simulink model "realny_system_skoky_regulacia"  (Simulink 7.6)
settings: Solver=ode4  StartTime=0.0  StopTime=150  FixedStep=0.2  RelTol=1e-3
undefined symbols (not defined in the file or in its folder): ABOVE_NORMAL_PRIORITY, COM3, D, I, lightbulb

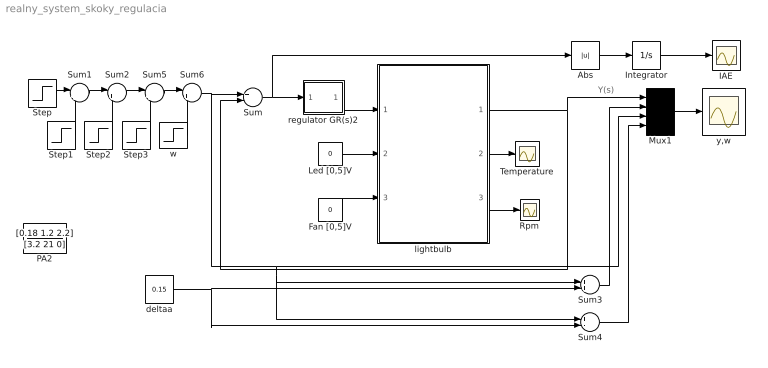
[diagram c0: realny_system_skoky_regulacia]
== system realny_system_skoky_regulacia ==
  note: Y(s)
  Abs : Abs
  Fan [0,5]V : Constant  Value=0
  IAE : Scope
  Integrator : Integrator
  Led [0,5]V : Constant  Value=0
  Mux1 : Mux
  PA2 : TransferFcn  Numerator=[0.18 1.2 2.2]  Denominator=[3.2 21 0]
  Rpm : Scope
  Step : Step  Time=0  After=11  SampleTime=0
  Step1 : Step  Time=30  After=30  SampleTime=0
  Step2 : Step  Time=60  After=-11  SampleTime=0
  Step3 : Step  Time=90  After=-25  SampleTime=0
  Sum : Sum  Inputs=+-
  Sum{1..2,5..6} (4 alike) : Sum  Inputs=|++
  Sum3 : Sum
  Sum4 : Sum  Inputs=+-
  Temperature : Scope
  deltaa : Constant  Value=0.15
  lightbulb : Subsystem  AncestorBlock=lightbulb/lightbulb
  regulator GR(s)2 : Subsystem  mask(PID Controller){P=0.059142,  I=0.059142/0.5163,  D=0}
      mask prompts: P "Proportional";  I "Integral";  D "Derivative"
      mask help: Enter expressions for proportional, integral, and derivative terms. P+I/s+Ds
  w : Step  Time=120  After=17  SampleTime=0
  y,w : Scope
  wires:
  Sum6/1 -> Sum3/1, Sum4/1, Mux1/3, Sum/1
  regulator GR(s)2/1(Out_1) -> lightbulb/1(bulb)
  Mux1/1 -> y,w/1
  deltaa/1 -> Sum3/2, Sum4/2
  Sum3/1 -> Mux1/2
  Sum4/1 -> Mux1/4
  lightbulb/1(light) -> Sum/2, Mux1/1
  Step1/1 -> Sum1/2
  Step/1 -> Sum1/1
  Step2/1 -> Sum2/2
  Step3/1 -> Sum5/2
  Sum2/1 -> Sum5/1
  Sum1/1 -> Sum2/1
  Sum5/1 -> Sum6/1
  w/1 -> Sum6/2
  Fan [0,5]V/1 -> lightbulb/3(fan)
  lightbulb/2(temperature) -> Temperature/1
  lightbulb/3(rpm) -> Rpm/1
  Led [0,5]V/1 -> lightbulb/2(led)
  Integrator/1 -> IAE/1
  Abs/1 -> Integrator/1
  Sum/1 -> regulator GR(s)2/1(In_1), Abs/1

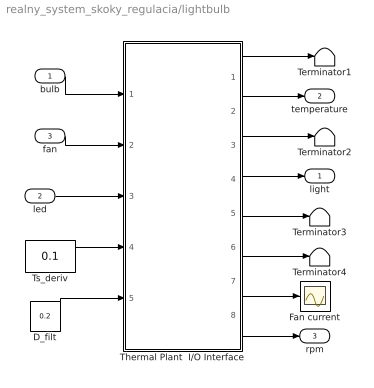
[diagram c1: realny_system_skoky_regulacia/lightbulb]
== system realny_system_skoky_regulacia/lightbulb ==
  bulb : Inport
  led : Inport  Port=2
  fan : Inport  Port=3
  D_filt : Constant  Value=0.2
  Fan current : Scope
  Terminator{1..4} (4 alike) : Terminator
  Thermal Plant  I/O Interface : Subsystem  mask{Ts=0.2}
      mask prompts: Ts "Sample time (s)"
      mask init:
      | set_param(bdroot,'FixedStep',num2str(Ts));
  Ts_deriv : Constant  Value=0.1
  light : Outport
  temperature : Outport  Port=2
  rpm : Outport  Port=3
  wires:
  bulb/1 -> Thermal Plant  I/O Interface/1(Bulb)
  Thermal Plant  I/O Interface/8(Fan rpm) -> rpm/1
  Thermal Plant  I/O Interface/7(Fan current) -> Fan current/1
  D_filt/1 -> Thermal Plant  I/O Interface/5(D_filt)
  Ts_deriv/1 -> Thermal Plant  I/O Interface/4(Ts_deriv)
  led/1 -> Thermal Plant  I/O Interface/3(LED)
  fan/1 -> Thermal Plant  I/O Interface/2(Fan)
  Thermal Plant  I/O Interface/1(Ambient temperature) -> Terminator1/1
  Thermal Plant  I/O Interface/6(Derivative  of light intensity) -> Terminator4/1
  Thermal Plant  I/O Interface/5(Filtered light intensity) -> Terminator3/1
  Thermal Plant  I/O Interface/4(Light intensity) -> light/1
  Thermal Plant  I/O Interface/2(Temperature) -> temperature/1
  Thermal Plant  I/O Interface/3(Filtered temperature) -> Terminator2/1

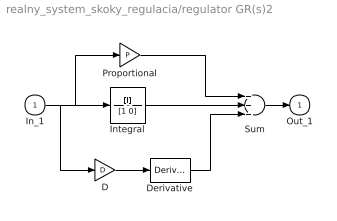
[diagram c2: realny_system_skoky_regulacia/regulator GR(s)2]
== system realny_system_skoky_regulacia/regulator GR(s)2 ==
  In_1 : Inport
  D : Gain  Gain=D
  Derivative : Derivative
  Integral : TransferFcn  Numerator=[I]  Denominator=[1 0]
  Proportional : Gain  Gain=P
  Sum : Sum  Inputs=+++
  Out_1 : Outport
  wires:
  Proportional/1 -> Sum/1
  Integral/1 -> Sum/2
  Derivative/1 -> Sum/3
  In_1/1 -> Integral/1, Proportional/1, D/1
  Sum/1 -> Out_1/1
  D/1 -> Derivative/1

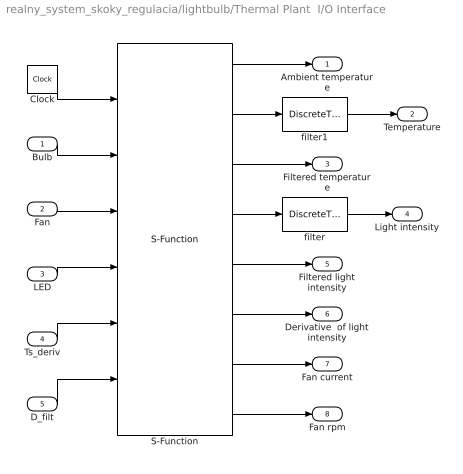
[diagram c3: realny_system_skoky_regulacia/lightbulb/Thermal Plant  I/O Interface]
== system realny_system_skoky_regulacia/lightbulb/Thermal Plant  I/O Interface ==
  Bulb : Inport
  Fan : Inport  Port=2
  LED : Inport  Port=3
  Ts_deriv : Inport  Port=4
  D_filt : Inport  Port=5
  Clock : Clock
  S-Function : S-Function  Priority=1  FunctionName=udaq28LT_v1R13  Parameters=com_port, Ts, events_ot, rd_timeout, matlab_prior, warning, printout  EnableBusSupport=off  mask(uDAQ28/LT Communication Interface){com_port=COM3, Ts=Ts, events_ot=1, rd_timeout=Ts/2*1000, matlab_prior=ABOVE_NORMAL_PRIORITY, warning=on, printout=off}
      mask prompts: com_port "Serial port:"; Ts "Sample time (sec):"; events_ot "Sampling delayed (%):"; rd_timeout "Read timeout (msec, lower than sample time):"; matlab_prior "Matlab priority"; warning "Warning if delayed (error if unchecked)"; printout "Detailed timing and timeout  printout"
      mask help: (c) 2006 Martin Kamensky Serial port - USB serial port number assigned to uDAQ28/LT system Sampling time (sec) - the lowest working value in Windows is about 0.04 - 0.05 s Sample delayed (%) - number of events (percentually) when simulink loop can take more than time determined by sample time Read timeout (msec) - timeout for reading data from the port (the lowest working value is about 25 ms) Matlab priority : NORMAL_PRIORITY - priority of common Windows application ABOVE_NORMAL_PRIORITY - recommended - higher priority than common Windows application priority HIGH_PRIORITY - recommended - hig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
      mask init:
      | %set_param(bdroot,'FixedStep',get_param(gcb,'Ts'));
      | set_param(bdroot,'Solver','ode4');
  filter : DiscreteTransferFcn  Numerator=0.6  Denominator=[1 -0.4]  SampleTime=Ts
  filter1 : DiscreteTransferFcn  Numerator=0.6  Denominator=[1 -0.4]  SampleTime=Ts
  Ambient temperature : Outport
  Temperature : Outport  Port=2
  Filtered temperature : Outport  Port=3
  Light intensity : Outport  Port=4
  Filtered light intensity : Outport  Port=5
  Derivative  of light intensity : Outport  Port=6
  Fan current : Outport  Port=7
  Fan rpm : Outport  Port=8
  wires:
  S-Function/8 -> Fan rpm/1
  S-Function/7 -> Fan current/1
  S-Function/6 -> Derivative  of light intensity/1
  S-Function/5 -> Filtered light intensity/1
  S-Function/4 -> filter/1
  S-Function/3 -> Filtered temperature/1
  S-Function/2 -> filter1/1
  S-Function/1 -> Ambient temperature/1
  D_filt/1 -> S-Function/6
  Ts_deriv/1 -> S-Function/5
  LED/1 -> S-Function/4
  Fan/1 -> S-Function/3
  Bulb/1 -> S-Function/2
  Clock/1 -> S-Function/1
  filter1/1 -> Temperature/1
  filter/1 -> Light intensity/1
